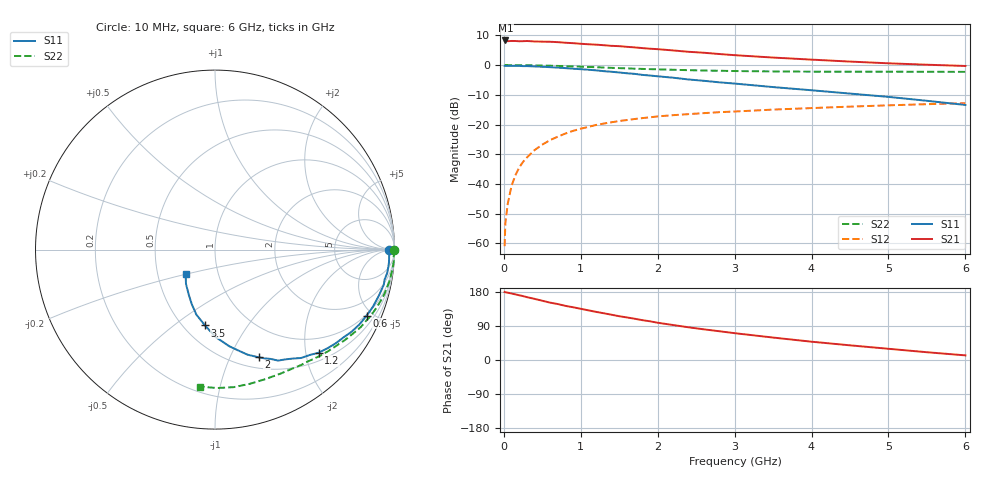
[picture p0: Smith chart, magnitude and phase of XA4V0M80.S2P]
! SIEMENS Discrete & RF Semiconductors
! BFY180
! Si NPN RF Bipolar Junction Transistor in MICRO-X
! VCE = 4 V  IC = 0.8 mA
! Common Emitter S-Parameters:  May  1997
# GHz  S  MA  R  50
!  f  S11  S21  S12  S22
! GHz  MAG  ANG  MAG  ANG  MAG  ANG  MAG  ANG
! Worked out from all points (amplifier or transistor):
!   36 points, 10 MHz to 6 GHz, reference 50 ohm
!   highest |S21| = 8.3 dB at 20 MHz (marker M1)
!   |S21| within 3 dB of that: start of sweep to 2.031 GHz
!   unconditionally stable (mu >= 1): 4.402 GHz to end of sweep
!   at 250 MHz: K = 0.07, MSG = 20.3 dB, |S12| = -32.5 dB
!   at 1.4 GHz: K = 0.45, MSG = 12.9 dB, |S12| = -19.2 dB
!   at 6 GHz: K = 1.04, MAG = 5.0 dB, |S12| = -12.8 dB
!   S11 on the Smith chart (normalised r, x): 10 MHz: 66, -8; 600 MHz: 0.95, -4.62; 1.2 GHz: 0.66, -2.26; 2 GHz: 0.62, -1.28; 3.5 GHz: 0.63, -0.65; 6 GHz: 0.70, -0.20
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0.01  0.9705 -0.2  2.541 179.6  0.0009 95.3  0.9974 -0.2
0.02  0.969 -0.8  2.592 178.8  0.0022 99.1  0.9999 -0.5
0.05  0.9708 -1.7  2.522 177.7  0.0046 87.4  0.9983 -1.3
0.1  0.972 -4.1  2.543 175.5  0.0093 86.9  0.9954 -2.5
0.15  0.9703 -6.0  2.539 173.2  0.014 85.4  0.9982 -3.8
0.2  0.9682 -7.8  2.513 170.8  0.0189 85.0  0.9961 -5.0
0.3  0.9606 -11.8  2.538 165.9  0.0279 81.3  0.9921 -7.5
0.4  0.948 -15.8  2.493 161.3  0.0372 78.8  0.9885 -9.9
0.6  0.9218 -23.5  2.465 151.4  0.0546 73.0  0.9755 -14.7
0.8  0.8882 -31.0  2.374 142.9  0.0705 67.5  0.9578 -19.4
1.1  0.8345 -41.1  2.235 131.0  0.0912 60.1  0.9284 -25.7
1.2  0.8142 -44.9  2.204 127.0  0.0984 57.8  0.9202 -27.9
1.5  0.7496 -54.0  2.078 115.5  0.1145 51.4  0.8882 -33.6
2  0.6471 -68.0  1.849 98.3  0.137 43.3  0.8472 -41.9
2.2  0.6128 -72.8  1.761 92.3  0.1436 40.1  0.8334 -45.1
2.4  0.5723 -77.6  1.672 86.3  0.1495 37.7  0.8197 -48.0
2.8  0.5126 -85.6  1.534 75.9  0.1613 33.2  0.8017 -53.4
3.5  0.4262 -97.5  1.337 59.2  0.1782 26.5  0.7812 -62.4
4  0.3768 -106.0  1.234 48.3  0.189 22.2  0.7742 -68.8
4.5  0.3314 -112.9  1.144 38.7  0.2 18.1  0.7726 -75.4
5.5  0.2505 -130.2  1.013 20.5  0.2199 10.1  0.7714 -89.1
6  0.2133 -140.1  0.965 12.2  0.2287 5.8  0.7678 -96.1
